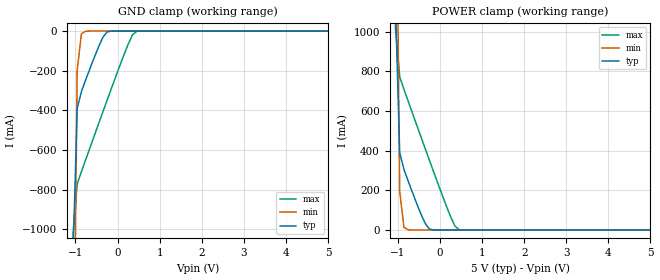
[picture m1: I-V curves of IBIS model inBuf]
| IBIS file created by T2B Version 15.0.2.03101 S001
| Cadence Design Systems, Inc. 2011
[IBIS ver] 4.0
[File name]  f2915.ibs
[File Rev]  0.1
[Date]   December 12, 2018
[Source] Integrated Device Technology, Inc.
[Notes] PVT : typ = TT 5.0v 25c
   min = SS 4.5v 105c
   max = FF 5.5v -40
[Disclaimer]
IDT hereby grants the user of this IBIS model a non-exclusive,
nontransferable license to use this IBIS model under the following terms.
Before using this IBIS model, the user should read this license.
If the user does not accept these terms,  the IBIS model should be
returned to IDT within 30 days.
   The user is granted this license only to use the IBIS model and
is not granted rights to sell, load, rent, lease or license the IBIS
model in whole or in part, or in modified form to anyone other than
user. User may modify the IBIS model to suit its specific
applications but rights to derivative works and such modifications
shall belong to IDT.
   This IBIS model is provided on an "AS IS" basis and IDT makes
absolutely no warranty with respect to the information contained
herein. IDT DISCLAIMS AND CUSTOMER WAIVES ALL WARRANTIES, EXPRESS
OR IMPLIED, INCLUDING WARRANTIES OF MERCHANTABILITY OR FITNESS FOR
A PARTICULAR PURPOSE. The entire risk as to quality and performance
is with the Customer. ACCORDINGLY, IN NO EVENT SHALL THE COMPANY BE
LIABLE FOR ANY DAMAGES, WHETHER IN CONTRACT OR TORT,INCLUDING ANY
LOST PROFITS OR OTHER INCIDENTAL, CONSEQUENTIAL, EXEMPLARY, OR
PUNITIVE DAMAGES ARISING OUT OF THE USE OR APPLICATION OF THE IBIS
model provided in this package. Further, IDT reserves the right to
make changes without notice to any product herein to improve
reliability, function, or design. IDT does not convey any license
under patent rights or any other intellectual property rights,
including those of third parties.
   IDT is not obligated to provide maintenance or support
for the licensed IBIS model.
[Copyright] Copyright 2015 by Integrated Device Technology, Inc.
|   Component f2915
[Component] f2915
[Manufacturer] Integrated Device Technology, Inc.
[Package]
| variable   typ   min   max
R_pkg   2.000m   1.000m   4.000m
L_pkg   0.200nH   0.100nH   0.400nH
C_pkg   2.000pF   1.000pF   4.000pF
[Pin]  signal_name   model_name   R_pin   L_pin   C_pin
in   in   inBuf
VDD   VDD   POWER
VGND   VGND   GND
| Models and submodels in the file (1): inBuf (Input)
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|   Model inBuf
[Model] inBuf
Model_type Input
Polarity   Non-Inverting
Vinl =  0.600V
Vinh =  1.100V
C_comp   0.521pF   0.500pF   0.528pF
C_comp_pullup   0.156pF   0.153pF   0.160pF
[Temperature Range]   25.000   0.105k   -40.000
[Voltage Range]   5.000V   4.500V   5.500V
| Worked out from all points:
|   GND clamp passes 1 mA (typ) near -0.17 V on its own axis
|   POWER clamp passes 1 mA (typ) near -0.17 V on its own axis
[GND_clamp]
|Voltage   I(typ)   I(min)   I(max)
-5V       -302.4A    -302.4A    -303A
-1.061V   -1.155A    -2.328A    -1.026A
-960mV    -389.9mA   -198.2mA   -771.7mA
-859mV    -305.1mA   -13.15mA   -709mA
-758mV    -246.6mA   -824.8uA   -649mA
-455mV    -80.78mA   -117.4nA   -469.9mA
-354mV    -33.45mA   -15.29nA   -410.6mA
-253mV    -4.685mA   -8.914nA   -351.4mA
252mV     -2.065nA   -3.525nA   -66.3mA
353mV     -1.63nA    -2.928nA   -19.91mA
454mV     -1.303nA   -2.428nA   -761.1uA
5V        0A         0A         0A
[POWER_clamp]
|Voltage   I(typ)   I(min)   I(max)
-5V       302.4A     302.4A     303A
-1.06V    1.132A     2.282A     1.018A
-959mV    388.4mA    193mA      771mA
-858mV    304.5mA    12.8mA     708.4mA
-757mV    246.1mA    802.3uA    648.5mA
-454mV    80.25mA    114.2nA    469.4mA
-353mV    33.04mA    15.13nA    410mA
-252mV    4.551mA    8.892nA    350.8mA
253mV     2.059nA    3.519nA    65.78mA
354mV     1.626nA    2.923nA    19.55mA
455mV     1.3nA      2.423nA    729uA
5V        0A         0A         0A
